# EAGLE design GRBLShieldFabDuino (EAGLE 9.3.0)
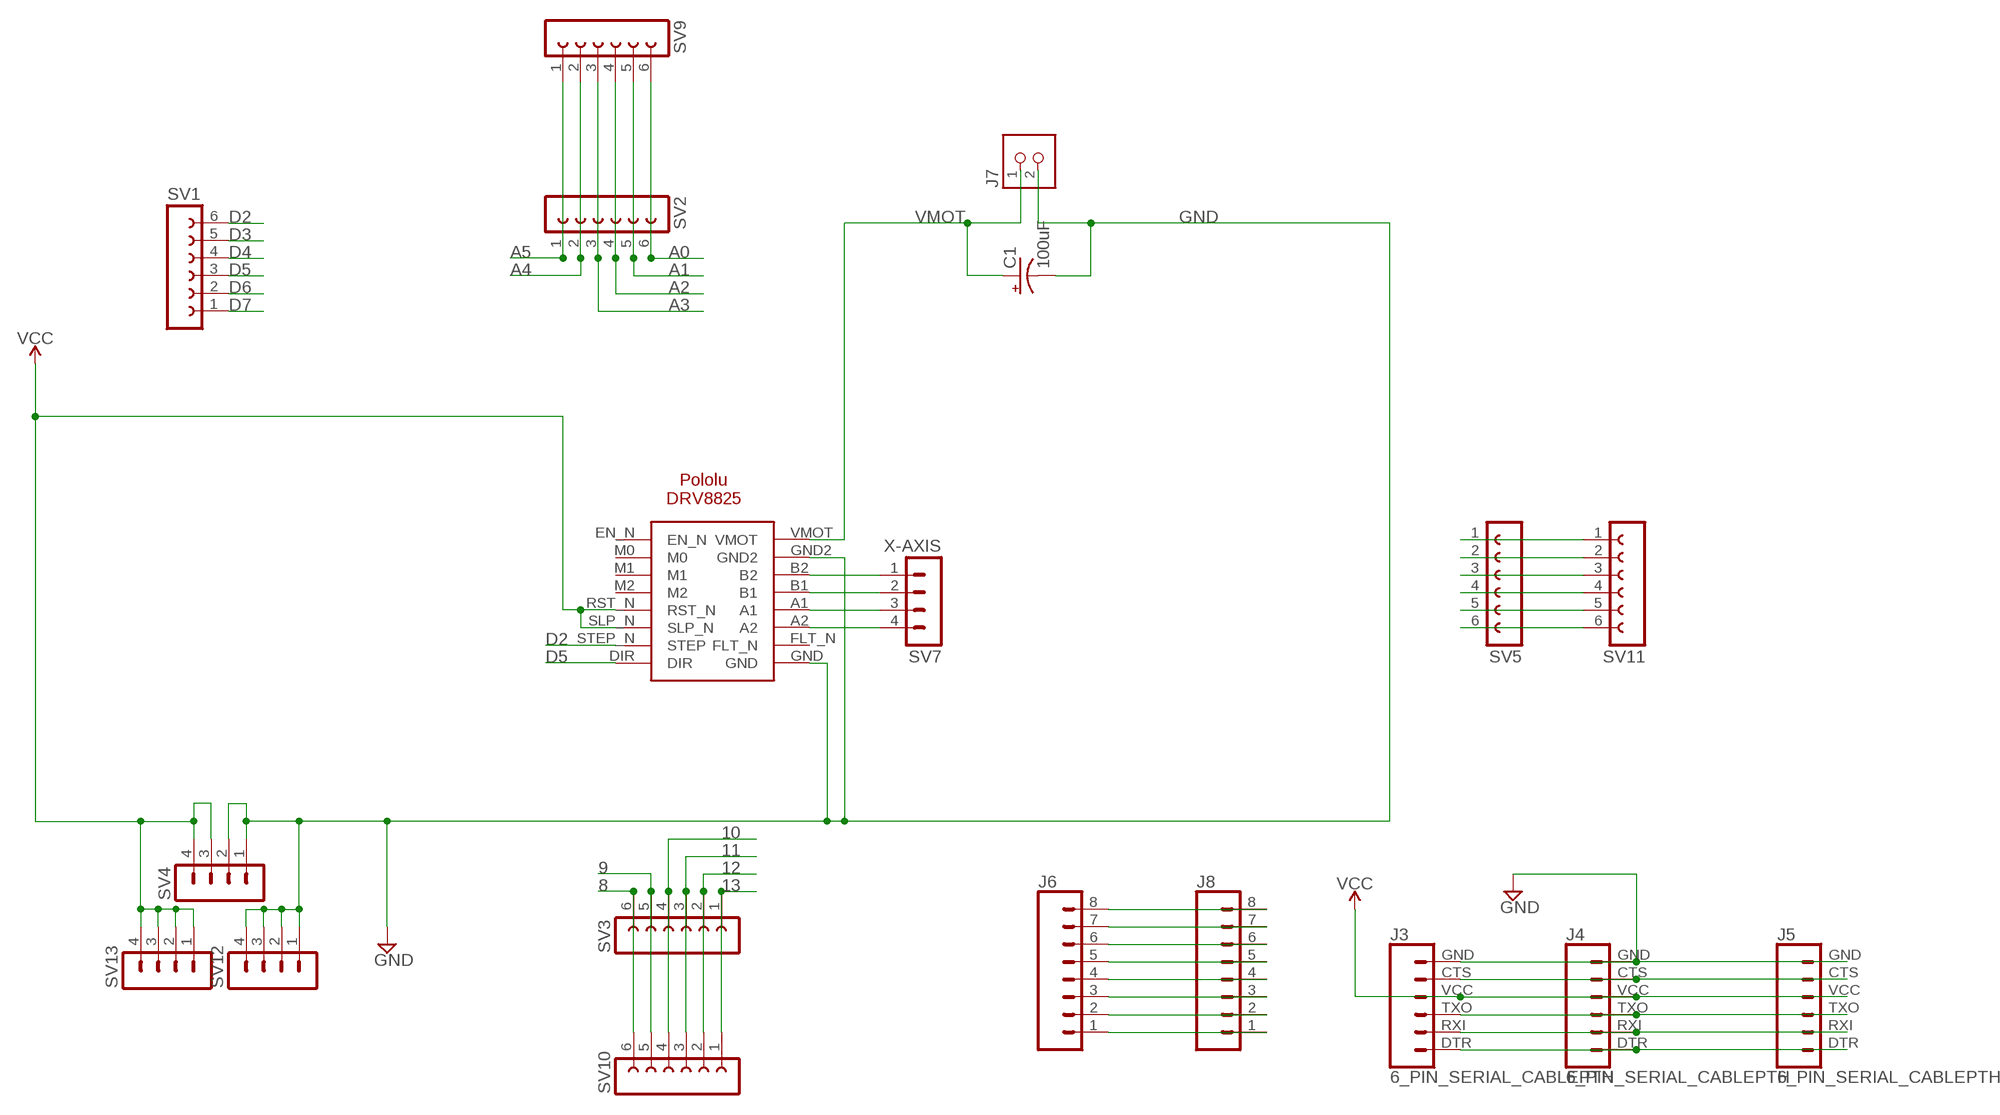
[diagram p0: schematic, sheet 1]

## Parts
C1  100uF  100UF-POLAR-RADIAL-2.5MM-25V-20%  [CPOL-RADIAL-2.5MM-6.5MM]
J3  6_PIN_SERIAL_CABLEPTH  [FTDI_BASIC]
J4  6_PIN_SERIAL_CABLEPTH  [FTDI_BASIC]
J5  6_PIN_SERIAL_CABLEPTH  [FTDI_BASIC]
J6  CONN_08"  [1X08]
J7  TERM-1X02-FABLAB  [ED555DS-2DS]
J8  CONN_08"  [1X08]
SV1  FE06-1  [FE06]
SV2  FE06-1  [FE06]
SV3  FE06-1  [FE06]
SV4  MA04-1  [MA04-1]
SV5  FE06-1  [FE06]
SV7  X-AXIS  MA04-1  [MA04-1]
SV9  FE06-1  [FE06]
SV10  FE06-1  [FE06]
SV11  FE06-1  [FE06]
SV12  MA04-1  [MA04-1]
SV13  MA04-1  [MA04-1]
X-AXIS  POLOLU-DRV8825  [POLOLU-DRV8825]

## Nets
8: SV3.6 SV10.6
9: SV3.5 SV10.5
10: SV3.4 SV10.4
11: SV3.3 SV10.3
12: SV3.2 SV10.2
13: SV3.1 SV10.1
A0: SV2.6 SV9.6
A1: SV2.5 SV9.5
A2: SV2.4 SV9.4
A3: SV2.3 SV9.3
A4: SV2.2 SV9.2
A5: SV2.1 SV9.1
D2: SV1.6 X-AXIS.STEP_N(STEP)
D3: SV1.5
D4: SV1.4
D5: SV1.3 X-AXIS.DIR
D6: SV1.2
D7: SV1.1
GND: C1.2(-) J3.GND J4.GND J5.GND J7.2 SV4.1 SV4.2 SV12.1 SV12.2 SV12.3 SV12.4 X-AXIS.GND X-AXIS.GND2
N$2: J3.CTS J4.CTS J5.CTS
N$4: J3.TXO J4.TXO J5.TXO
N$5: SV7.1 X-AXIS.B2
N$6: SV7.2 X-AXIS.B1
N$7: SV7.3 X-AXIS.A1
N$8: SV7.4 X-AXIS.A2
N$9: J3.RXI J4.RXI J5.RXI
N$10: J3.DTR J4.DTR J5.DTR
N$11: J6.8 J8.8
N$13: SV5.1 SV11.1
N$14: SV5.2 SV11.2
N$15: SV5.3 SV11.3
N$16: SV5.4 SV11.4
N$17: SV5.5 SV11.5
N$18: SV5.6 SV11.6
N$26: J6.7 J8.7
N$27: J6.6 J8.6
N$28: J6.5 J8.5
N$29: J6.4 J8.4
N$30: J6.3 J8.3
N$31: J6.2 J8.2
N$32: J6.1 J8.1
VCC: J3.VCC J4.VCC J5.VCC SV4.3 SV4.4 SV13.1 SV13.2 SV13.3 SV13.4 X-AXIS.RST_N X-AXIS.SLP_N
VMOT: C1.1(+) J7.1 X-AXIS.VMOT
Unconnected: X-AXIS.EN_N X-AXIS.FLT_N X-AXIS.M0 X-AXIS.M1 X-AXIS.M2

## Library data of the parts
C1 = SparkFun-Capacitors:100UF-POLAR: 100µF polarized capacitors; PROD_ID: CAP-08439
J3-J5 = SparkFun-Connectors:6_PIN_SERIAL_CABLE: 6-pin header connection for use with the "FTDI BASIC" pinout - CABLE SIDE. Also known as "Arduino Serial Program Header". This is used on a design to provide a 6-pin connection point for serial communication usually from a USB cable (D+/D-) to these headers (RX/TX). It also has the remaining pins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
J6 J8 = SparkFun-Connectors:CONN_08: Multi connection point. Often used as Generic Header-pin footprint for 0.1 inch spaced/style header connections On any of the 0.1 inch spaced packages, you can populate with these: Break Away Headers - Straight (PRT-00116) Break Away Male Headers - Right Angle (PRT-00553) Female Headers (PRT-00115)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; PROD_ID: CONN-08438
J7 = fab:TERM-1X02: 3.5mm terminal block, 2 positions ED555-2DS as found in the fablab inventory.
SV1-SV3 SV5 SV9-SV11 = con-lsta:FE06-1: FEMALE HEADER; OC_FARNELL: unknown; OC_NEWARK: unknown
SV4 SV7 SV12 SV13 = con-lstb:MA04-1: PIN HEADER; OC_FARNELL: unknown; OC_NEWARK: unknown
X-AXIS = alvarop-lib:POLOLU-DRV8825

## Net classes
0 default: clearance 0.406 mm

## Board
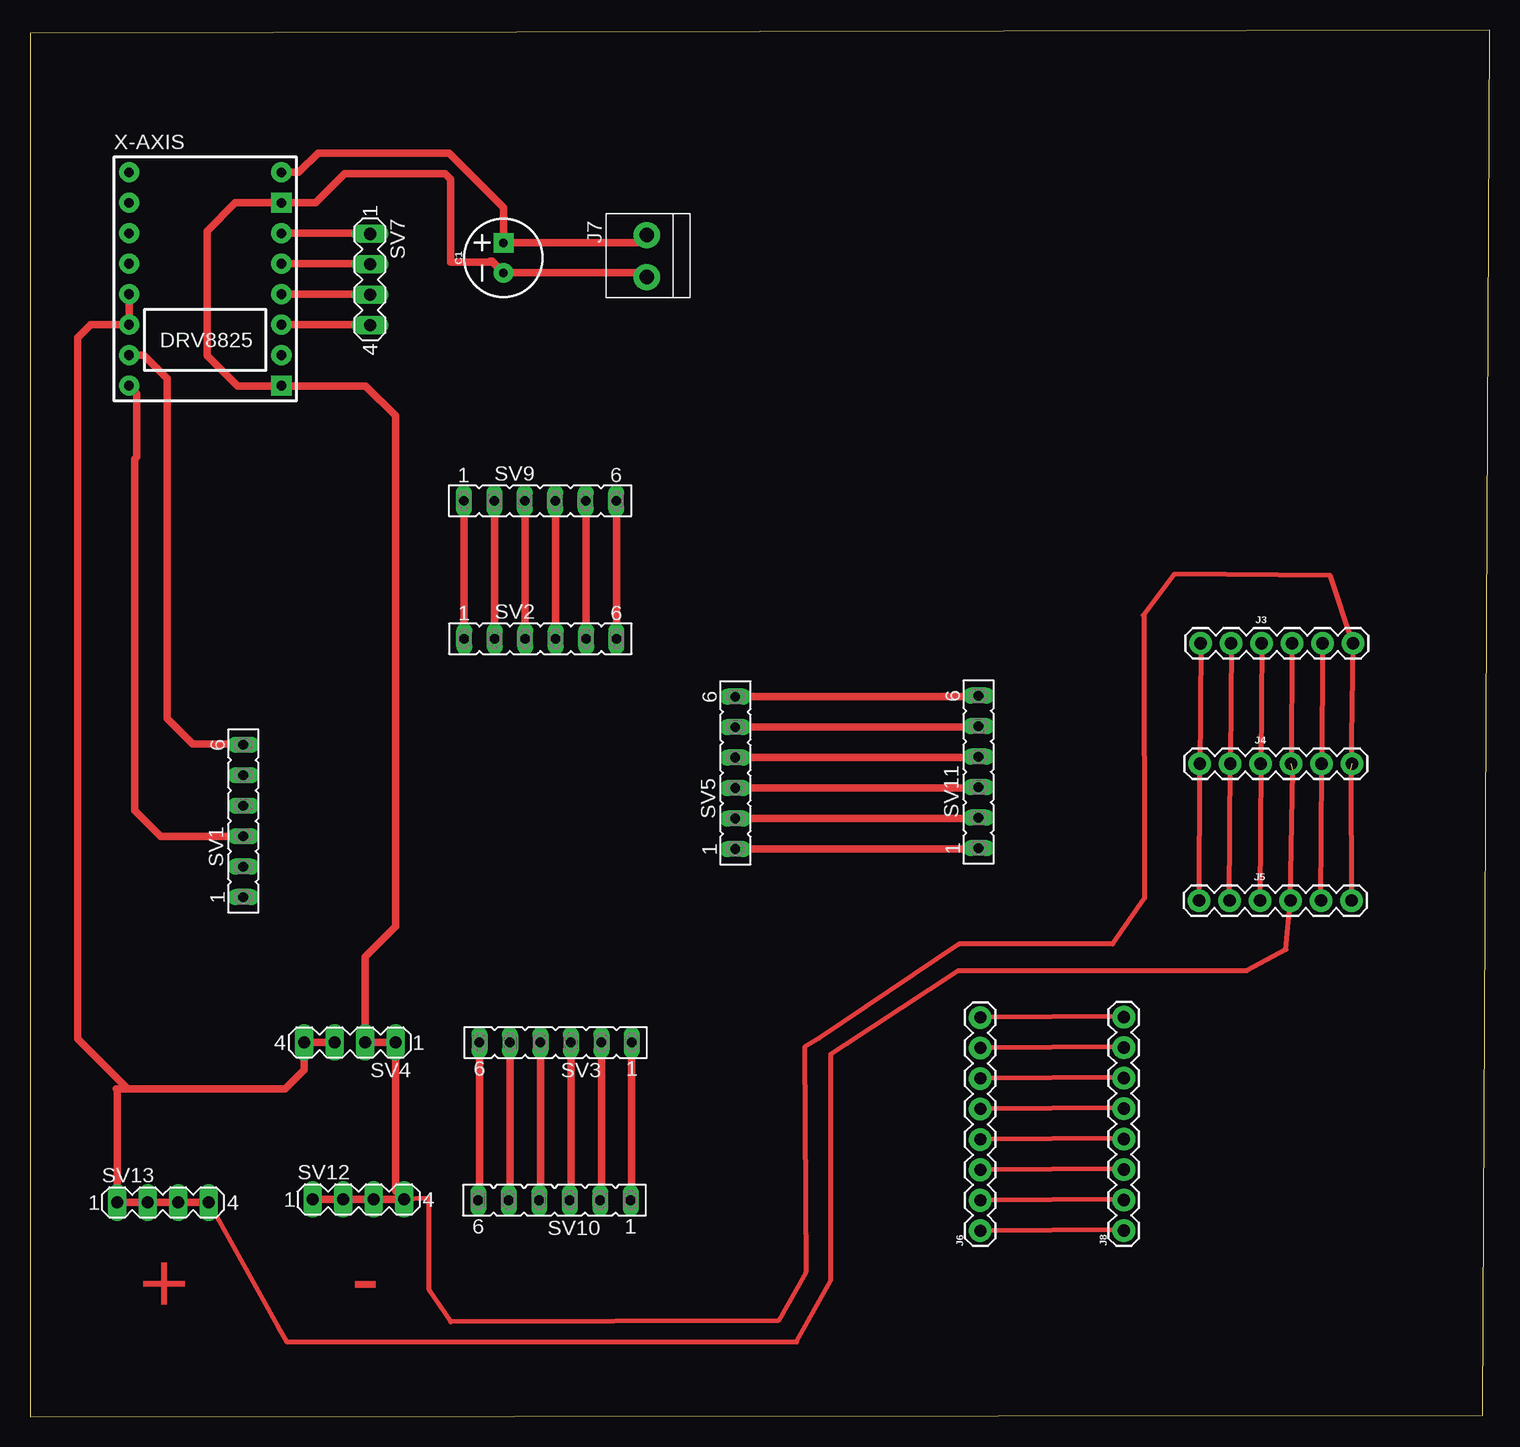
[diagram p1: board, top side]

Size 121.67 x 115.62 mm. Coordinates in mm from the lower left corner, seen from the top.
Outline: 0.03,0 121.09,0.13 121.67,115.62 0,115.34 0.03,0
Copper layers (1*16): Top 0.035mm / dielectric 1.5mm / Bottom 0.035mm
Design rules "default": minimum track width 6mil, minimum drill 0.35mm, track to track 6mil, track to pad 6mil, pad to pad 6mil, via to via 6mil, smd to smd 6mil, copper to edge 40mil, drill to drill 6mil, minimum pad ring 10mil, minimum via ring 8mil, stop-mask expansion 4mil, vias tented up to drill 0mil, thermal gap 10mil

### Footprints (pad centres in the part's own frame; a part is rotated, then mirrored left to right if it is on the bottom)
CPOL-RADIAL-2.5MM-6.5MM = drill 0.7 pad 1.651 square: 1 1.25,0 | drill 0.7 pad 1.651: 2 -1.25,0
FTDI_BASIC = drill 1.016 pad 1.88: CTS 10.16,0; DTR 0,0; GND 12.7,0; RXI 2.54,0; TXO 5.08,0; VCC 7.62,0
1X08 = drill 1.016 pad 1.88: 1 0,0; 2 2.54,0; 3 5.08,0; 4 7.62,0; 5 10.16,0; 6 12.7,0; 7 15.24,0; 8 17.78,0
ED555DS-2DS = drill 1.2 pad 2.184: 1 1.8,0; 2 -1.7,0
FE06 = drill 0.813 long: 1 -6.35,0; 2 -3.81,0; 3 -1.27,0; 4 1.27,0; 5 3.81,0; 6 6.35,0
MA04-1 = drill 1.016 long: 1 -3.81,0; 2 -1.27,0; 3 1.27,0; 4 3.81,0
POLOLU-DRV8825 = drill 0.8 pad 1.676: A1 6.35,-1.27; A2 6.35,-3.81; B1 6.35,1.27; B2 6.35,3.81; DIR -6.35,-8.89; EN_N -6.35,8.89; FLT_N 6.35,-6.35; M0 -6.35,6.35; M1 -6.35,3.81; M2 -6.35,1.27; RST_N -6.35,-1.27; SLP_N -6.35,-3.81; STEP_N -6.35,-6.35; VMOT 6.35,8.89 | drill 0.8 pad 1.676 square: GND 6.35,-8.89; GND2 6.35,6.35

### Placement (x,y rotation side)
C1  39.47,96.62 90 top
J3  97.59,64.49 0 top
J4  97.51,54.46 0 top
J5  97.46,43.05 0 top
J6  79.22,15.52 90 top
J7  51.41,96.72 90 top
J8  91.19,15.54 90 top
SV1  17.78,49.68 90 top
SV2  42.55,64.87 0 top
SV3  43.81,31.22 180 top
SV4  26.67,31.22 180 top
SV5  58.8,53.7 90 top
SV7  28.35,94.82 270 top
SV9  42.52,76.38 0 top
SV10  43.71,18.06 180 top
SV11  79.07,53.77 90 top
SV12  27.38,18.14 0 top
SV13  11.07,17.88 0 top
X-AXIS  14.61,94.87 0 top

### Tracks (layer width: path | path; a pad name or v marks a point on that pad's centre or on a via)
8
  Top 0.61: SV3.6 37.47,18.16 SV10.6
9
  Top 0.61: SV3.5 40.01,18.16 SV10.5
10
  Top 0.61: SV3.4 42.55,18.16 SV10.4
11
  Top 0.61: SV3.3 45.09,18.16 SV10.3
12
  Top 0.61: SV3.2 47.63,18.16 SV10.2
13
  Top 0.61: SV3.1 50.17,18.16 SV10.1
A0
  Top 0.61: SV2.6 48.9,76.35 SV9.6
A1
  Top 0.61: SV2.5 46.36,76.35 SV9.5
A2
  Top 0.61: SV2.4 43.82,76.35 SV9.4
A3
  Top 0.61: SV2.3 41.28,76.35 SV9.3
A4
  Top 0.61: SV2.2 38.74,76.35 SV9.2
A5
  Top 0.61: SV2.1 36.2,76.35 SV9.1
D2
  Top 0.61: X-AXIS.STEP_N 9.47,88.52 11.43,86.56 11.43,58.22 13.56,56.08 17.73,56.08 SV1.6
D5
  Top 0.61: X-AXIS.DIR 8.92,85.32 8.92,80.01 8.74,79.83 8.74,50.57 10.9,48.41 SV1.3
GND  (1 unrouted)
  Top 0.406: J5.GND 110.08,53.95 J3.GND 108.38,70.15 95.4,70.26 92.87,66.91 | 92.87,66.91 92.81,66.83 | 92.87,66.91 92.91,43.26 90.25,39.42 77.44,39.42 65.81,31.6 64.57,30.84 64.67,12.04 62.38,8.03 35.1,7.92 33.27,10.59 33.27,18.24 30.89,18.14
  Top 0.61: 20.93,85.95 17.3,85.95 14.76,88.49 14.76,98.86 17.12,101.22 X-AXIS.GND2 23.83,101.22 26.24,103.63 34.62,103.63 35.08,103.17 35.08,96.27 38.58,96.27 C1.2 | 20.93,85.95 X-AXIS.GND | SV12.1 SV12.2 SV12.3 30.89,18.14 SV12.4 30.48,18.85 SV4.1 SV4.2 27.94,38.35 30.48,40.89 30.48,83.46 27.99,85.95 20.93,85.95 | C1.2 51.06,95.37 J7.2 | C1.2 38.51,96.34 38.35,96.34
N$2
  Top 0.406: J5.CTS 107.67,54.08 | 107.67,54.08 J4.CTS | J3.CTS 107.67,54.08
N$4
  Top 0.406: J3.TXO J4.TXO J5.TXO
N$5
  Top 0.61: X-AXIS.B2 28.3,98.68 SV7.1
N$6
  Top 0.61: X-AXIS.B1 28.3,96.14 SV7.2
N$7
  Top 0.61: X-AXIS.A1 28.3,93.6 SV7.3
N$8
  Top 0.61: X-AXIS.A2 28.3,91.06 SV7.4
N$9
  Top 0.406: J3.RXI 100.05,54.64 | 100.05,54.64 J4.RXI | J5.RXI 100.05,54.64
N$10
  Top 0.406: J5.DTR 97.51,53.8 | 97.51,53.8 J4.DTR | J3.DTR 97.51,53.8
N$11
  Top 0.406: J8.8 91.13,33.38 J6.8
N$13
  Top 0.61: SV5.1 78.99,47.35 SV11.1
N$14
  Top 0.61: SV5.2 78.99,49.89 SV11.2
N$15
  Top 0.61: SV5.3 78.99,52.43 SV11.3
N$16
  Top 0.61: SV5.4 78.99,54.97 SV11.4
N$17
  Top 0.61: SV5.5 78.99,57.51 SV11.5
N$18
  Top 0.61: SV5.6 78.99,60.05 SV11.6
N$26
  Top 0.406: J8.7 91.13,30.84 J6.7
N$27
  Top 0.406: J8.6 91.13,28.3 J6.6
N$28
  Top 0.406: J8.5 91.13,25.76 J6.5
N$29
  Top 0.406: J8.4 91.13,23.22 J6.4
N$30
  Top 0.406: J8.3 91.13,20.68 J6.3
N$31
  Top 0.406: J8.2 91.13,18.14 J6.2
N$32
  Top 0.406: J8.1 91.13,15.6 J6.1
VCC  (1 unrouted)
  Top 0.406: J3.VCC J4.VCC | 105.28,53.95 J5.VCC 104.7,38.96 101.45,37.21 77.39,37.21 66.75,30.25 66.75,11.4 63.91,6.25 21.39,6.27 20.67,7.56 SV13.4
  Top 0.61: SV4.3 SV4.4 22.86,28.93 21.26,27.33 8.15,27.33 | X-AXIS.SLP_N X-AXIS.RST_N | X-AXIS.SLP_N 8.38,90.93 | X-AXIS.SLP_N 5.05,91.06 3.96,89.97 3.96,31.52 8.15,27.33 | 8.15,27.33 7.19,27.33 7.26,27.25 SV13.1 SV13.2 SV13.3 SV13.4
VMOT
  Top 0.61: X-AXIS.VMOT 22.4,103.76 24,105.36 34.93,105.36 39.47,100.81 C1.1 | 39.28,98.06 C1.1 | C1.1 50.76,97.87 J7.1

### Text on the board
Top: - | +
